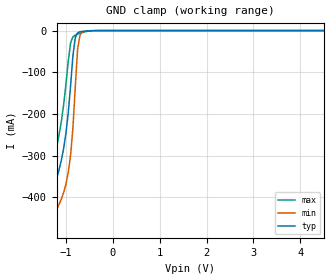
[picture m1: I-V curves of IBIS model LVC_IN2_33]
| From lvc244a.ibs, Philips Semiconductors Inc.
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|   Model LVC_IN2_33
[Model]   LVC_IN2_33
Model_type   Input
Vinl =   0.8000V
Vinh =   2.0000V
C_comp   2.78pF   1.99pF   3.72pF
[Model Spec]
| Note: The input and output voltage ratings may be exceeded if the input and
|   output current ratings are observed (please refer to the data sheet)
|   Subparameter   typ   min   max
| Thresholds
Vinh   2.0   NA   NA
Vinl   0.8   NA   NA
| Overshoot
S_overshoot_high   6.5   6.5   6.5   | Static overshoot
S_overshoot_low   -0.5   -0.5   -0.5
D_overshoot_high   7.2   7.2   7.2   | Dynamic overshoot
D_overshoot_low   -0.95   -0.9   -1.0
D_overshoot_time   3n   3n   3n
|Ambient temperature:   25.0000   85.0000   -40.0000
[Temperature Range]   40.0000   100.0000   -25.0000
[Voltage Range]   3.3000V   3.0000V   3.6000V
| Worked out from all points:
|   GND clamp passes 1 mA (typ) near -0.57 V on its own axis
|Process Range   nominal   slow   fast
[GND_clamp]
| voltage   I(typ)   I(min)   I(max)
-5.5V     -4.567A    -4.624A    -4.51A
-1.45V    -555.2mA   -621.5mA   -488.4mA
-1.35V    -461.8mA   -528.7mA   -394.3mA
-1.3V     -417.5mA   -485mA     -349.4mA
-1.1V     -312.4mA   -404.8mA   -219.8mA
-950mV    -197.3mA   -340.4mA   -73.13mA
-900mV    -132mA     -298.5mA   -29.44mA
-850mV    -59.79mA   -233mA     -14.94mA
-800mV    -16.87mA   -135mA     -10.93mA
-750mV    -5.479mA   -44.49mA   -8.487mA
-700mV    -2.88mA    -11.01mA   -6.407mA
5.5V      1.567nA    9.324nA    202.5pA
